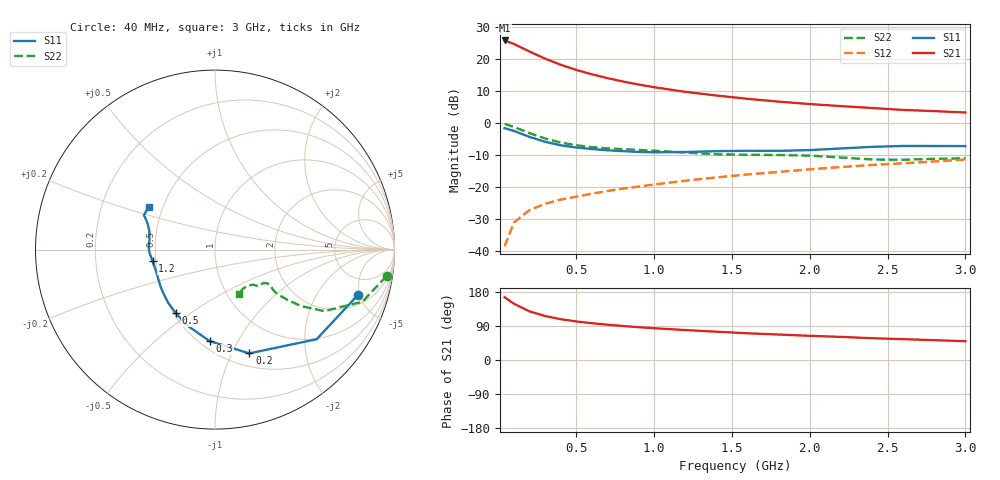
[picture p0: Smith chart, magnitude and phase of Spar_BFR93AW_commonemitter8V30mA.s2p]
! Filename:  BFR93AWH.S2P  Version:  4.0
! NXP part #: BFR93AW  Date: Jun 1994
! Bias condition: Vce=8V, Ic=30mA
#  MHz  S  MA  R  50
! Freq  S11  S21  S12  S22  !GUM [dB]
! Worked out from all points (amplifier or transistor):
!   21 points, 40 MHz to 3 GHz, reference 50 ohm
!   highest |S21| = 25.8 dB at 40 MHz (marker M1)
!   |S21| within 3 dB of that: start of sweep to 180.9 MHz
!   unconditionally stable (mu >= 1): 919.8 MHz to end of sweep
!   at 300 MHz: K = 0.58, MSG = 22.7 dB, |S12| = -25.2 dB
!   at 1 GHz: K = 1.02, MAG = 14.2 dB, |S12| = -19.2 dB
!   at 3 GHz: K = 1.04, MAG = 6.2 dB, |S12| = -11.4 dB
!   lowest NFmin = 2.10 dB at 500 MHz
!   S11 on the Smith chart (normalised r, x): 40 MHz: 2.85, -4.78; 200 MHz: 0.64, -1.17; 300 MHz: 0.56, -0.77; 500 MHz: 0.51, -0.44; 1.2 GHz: 0.48, -0.07; 3 GHz: 0.42, +0.25
40  0.835 -17.7  19.5 165.7  0.012 80.3  0.967 -8.8
100  0.755 -41.4  17.19 148.4  0.028 69.7  0.871 -19.5
200  0.609 -71.7  13.11 128.4  0.044 60.1  0.698 -29.4
300  0.511 -93.3  10.14 116.1  0.055 56.2  0.575 -33.2
400  0.451 -109.6  8.143 107.7  0.064 56.1  0.498 -34.7
500  0.416 -121.7  6.762 101.8  0.071 56.9  0.451 -35.2
600  0.394 -131.7  5.781 97.1  0.079 58.4  0.422 -35.4
700  0.377 -139.7  5.04 93.2  0.087 59.7  0.404 -35.1
800  0.365 -146.7  4.464 89.7  0.095 61.2  0.392 -34.6
900  0.355 -153.3  4.005 86.6  0.102 62.3  0.382 -33.9
1000  0.35 -159.2  3.634 83.9  0.11 63.3  0.371 -33.2
1200  0.354 -169.6  3.077 79.0  0.126 65.0  0.347 -32.8
1400  0.365 -177.1  2.698 74.7  0.142 66.3  0.327 -34.7
1600  0.37 177.2  2.397 70.5  0.158 66.8  0.32 -38.2
1800  0.369 171.5  2.164 67.2  0.173 67.8  0.318 -39.9
2000  0.379 164.5  1.984 63.8  0.19 68.6  0.311 -40.6
2200  0.402 159.0  1.842 61.0  0.206 69.1  0.29 -42.4
2400  0.426 155.6  1.722 57.5  0.222 69.4  0.271 -47.8
2600  0.44 154.2  1.605 55.0  0.236 69.3  0.268 -55.0
2800  0.439 151.2  1.54 52.3  0.252 69.7  0.277 -59.6
3000  0.438 146.8  1.464 49.6  0.27 69.7  0.282 -62.1
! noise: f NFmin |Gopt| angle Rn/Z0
500  2.1  0.178  37.4  0.231
1000  2.6  0.193  144.2  0.32
2000  3.6  0.509  -154.2  0.22
